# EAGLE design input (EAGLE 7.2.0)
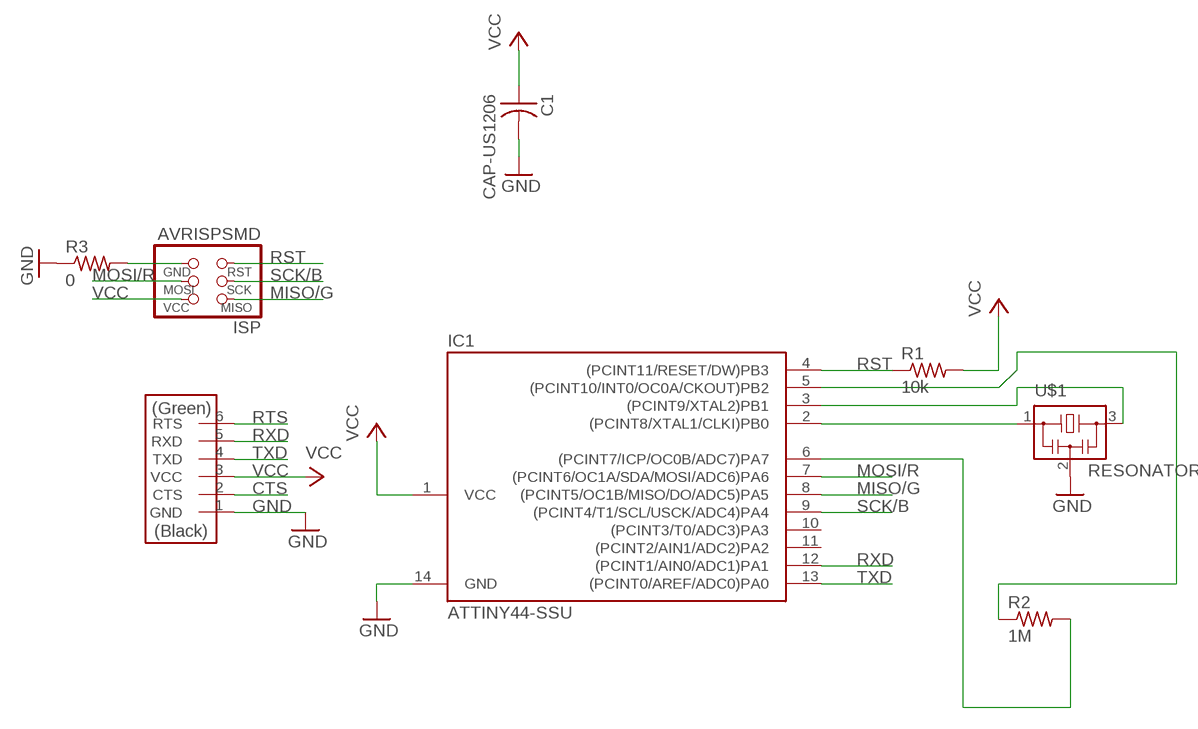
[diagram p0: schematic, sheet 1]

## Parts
C1  CAP-US1206  [C1206]
IC1  ATTINY44-SSU  [SOIC14]
ISP  AVRISPSMD  [2X03SMD]
R1  10k  RES-US1206  [R1206]
R2  1M  RES-US1206  [R1206]
R3  0  RES-US1206  [R1206]
U$1  RESONATOR  [EFOBM]
U$2  FTDI-SMD-HEADER  [1X06SMD]

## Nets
CTS: U$2.2(CTS)
GND: C1.2 IC1.14(GND) R3.1 U$1.2 U$2.1(GND)
MISO/G: IC1.8((PCINT5/OC1B/MISO/DO/ADC5)PA5) ISP.1(MISO)
MOSI/R: IC1.7((PCINT6/OC1A/SDA/MOSI/ADC6)PA6) ISP.4(MOSI)
N$1: IC1.5((PCINT10/INT0/OC0A/CKOUT)PB2) R2.1
N$2: IC1.6((PCINT7/ICP/OC0B/ADC7)PA7) R2.2
N$3: ISP.6(GND) R3.2
N$9: IC1.2((PCINT8/XTAL1/CLKI)PB0) U$1.1
N$10: IC1.3((PCINT9/XTAL2)PB1) U$1.3
RST: IC1.4((PCINT11/RESET/DW)PB3) ISP.5(RST) R1.1
RTS: U$2.6(RTS)
RXD: IC1.12((PCINT1/AIN0/ADC1)PA1) U$2.5(RXD)
SCK/B: IC1.9((PCINT4/T1/SCL/USCK/ADC4)PA4) ISP.3(SCK)
TXD: IC1.13((PCINT0/AREF/ADC0)PA0) U$2.4(TXD)
VCC: C1.1 IC1.1(VCC) ISP.2(VCC) R1.2 U$2.3(VCC)
Unconnected: IC1.10((PCINT3/T0/ADC3)PA3) IC1.11((PCINT2/AIN1/ADC2)PA2)

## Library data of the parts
C1 = fab:CAP-US
IC1 = fab:ATTINY44
ISP = fab:AVRISP
R1-R3 = fab:RES-US: Resistor (US Symbol)
U$1 = fab:RESONATOR
U$2 = fab:FTDI-SMD-HEADER

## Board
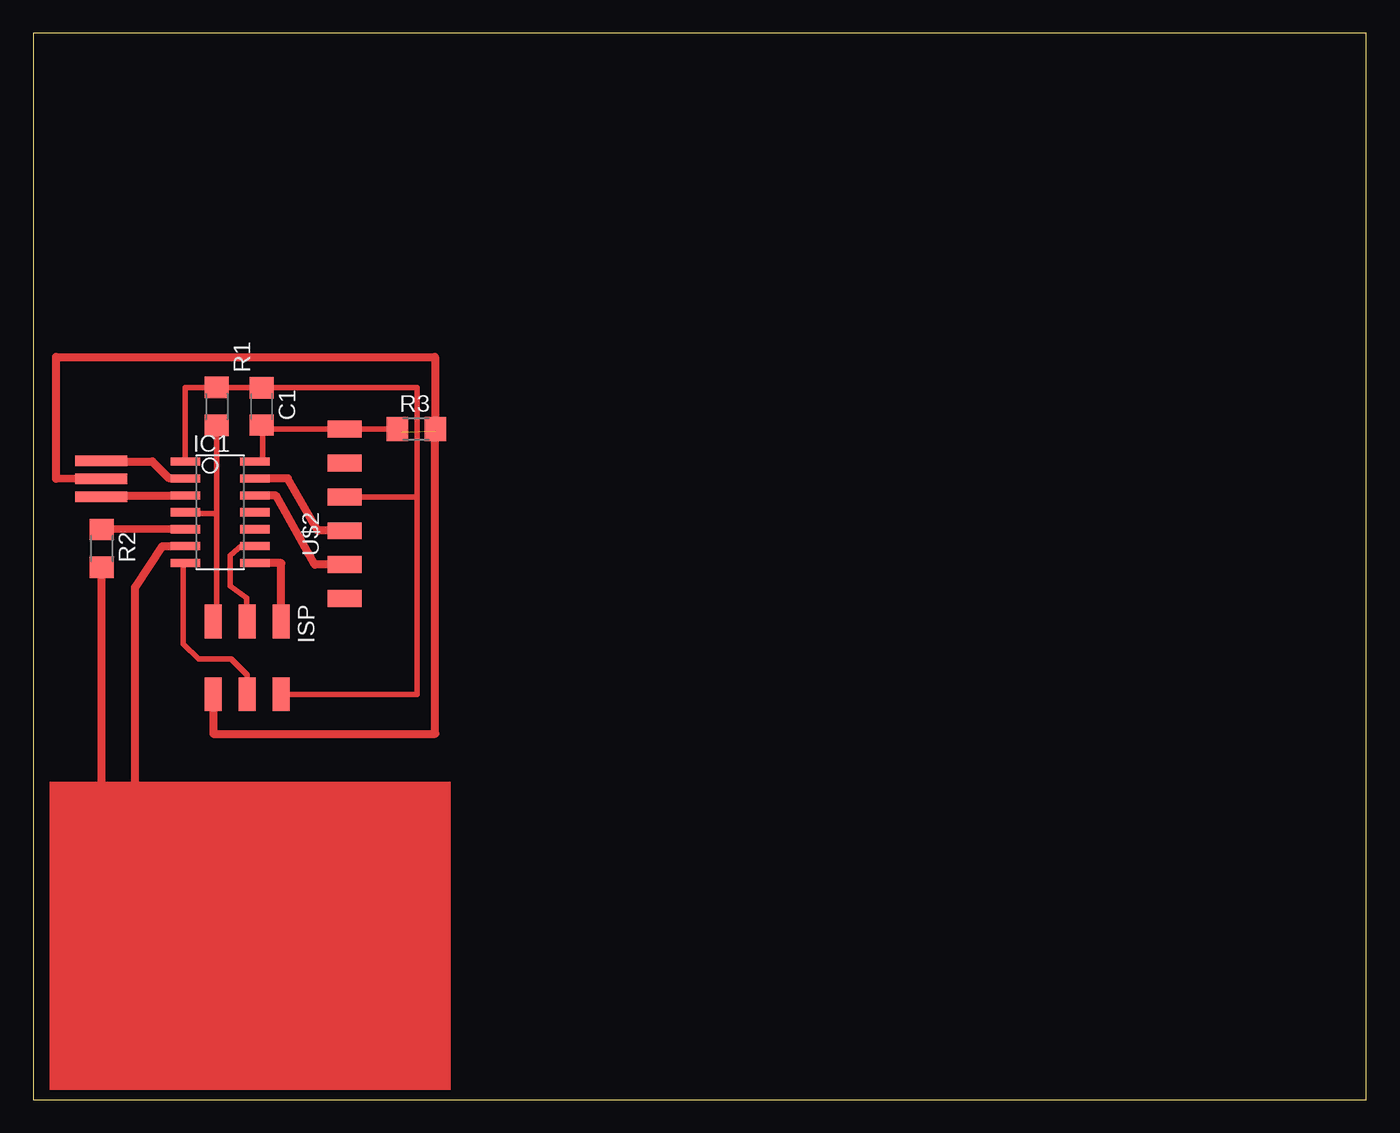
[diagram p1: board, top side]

Size 100 x 80 mm. Coordinates in mm from the lower left corner, seen from the top.
Outline: 0,0 100,0 100,80 0,80 0,0
Copper layers 1+16: Top 0.035mm / dielectric 1.5mm / Bottom 0.035mm
Design rules "fablab_17mils": minimum track width 10mil, minimum drill 0.8mm, track to track 17mil, track to pad 17mil, pad to pad 17mil, via to via 17mil, smd to smd 17mil, copper to edge 16mil, drill to drill 16mil, minimum pad ring 0.8mm, minimum via ring 0.8mm, stop-mask expansion 4mil, vias tented up to drill 0mil, thermal gap 1mm

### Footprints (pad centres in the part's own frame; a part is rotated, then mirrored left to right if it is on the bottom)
C1206 = smd 1.6 x 1.8: 1 -1.4,0; 2 1.4,0
SOIC14 = smd 0.61 x 2.21: 1 -3.81,-2.603; 2 -2.54,-2.603; 3 -1.27,-2.603; 4 0,-2.603; 5 1.27,-2.603; 6 2.54,-2.603; 7 3.81,-2.603; 8 3.81,2.603; 9 2.54,2.603; 10 1.27,2.603; 11 0,2.603; 12 -1.27,2.603; 13 -2.54,2.603; 14 -3.81,2.603
2X03SMD = smd 2.54 x 1.27: 1 -2.54,2.54; 2 2.92,2.54; 3 -2.54,0; 4 2.92,0; 5 -2.54,-2.54; 6 2.92,-2.54
R1206 = smd 1.6 x 1.803: 1 -1.422,0; 2 1.422,0
EFOBM = smd 0.8 x 3.9: 1 -1.35,0; 2 0,0; 3 1.35,0
1X06SMD = smd 2.54 x 1.27: 1 0,6.35; 2 0,3.81; 3 0,1.27; 4 0,-1.27; 5 0,-3.81; 6 0,-6.35

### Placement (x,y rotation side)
C1  17.15,52 270 top
IC1  14.02,44.06 270 top
ISP  16.05,33.33 270 top
R1  13.76,52.01 90 top
R2  5.14,41.35 270 top
R3  28.73,50.3 0 top
U$1  5.08,46.58 270 top
U$2  23.36,43.95 0 top

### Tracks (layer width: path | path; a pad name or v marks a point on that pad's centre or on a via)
GND  (1 unrouted)
  Top 0.406: C1.2 17.19,50.55 | 17.19,50.55 17.19,47.86 17.18,47.87 IC1.14 | 17.19,50.55 17.45,50.3 U$2.1 26.78,50.3 R3.1 27.64,50.09
  Top 0.61: U$1.2 1.71,46.56 1.71,55.71 30.14,55.72 30.14,50.14
MISO/G
  Top 0.406: 17.5,40.25 IC1.8
  Top 0.61: ISP.1 18.59,40.25 17.5,40.25
MOSI/R
  Top 0.406: IC1.7 11.26,40.1 11.26,34.19 12.39,33.06 14.86,33.06 16.05,31.87 ISP.4
N$1
  Top 0.61: IC1.5 R2.1
N$2
  Top 0.406: 7.67,38.47 7.62,38.43 | 7.62,22.23 5.08,22.23 5.14,22.29
  Top 0.61: 7.67,38.47 9.7,41.52 IC1.6 | 7.62,38.43 7.62,22.23 | 5.14,22.29 R2.2
N$3
  Top 0.406: ISP.6
  Top 0.61: ISP.6 13.51,27.44 30.15,27.44 R3.2
N$9
  Top 0.406: U$1.1 6.48,47.87 | 10.21,46.6 IC1.2
  Top 0.61: 6.48,47.87 8.94,47.87 10.21,46.6
N$10
  Top 0.406: U$1.3 6.48,45.33
  Top 0.61: 6.48,45.33 IC1.3
RST
  Top 0.406: R1.1 13.76,43.97 | 13.76,43.97 13.77,35.92 ISP.5 | IC1.4 11.41,43.98 13.76,43.97
RXD
  Top 0.61: U$2.5 21.11,40.14 18.22,45.31 IC1.12
SCK/B
  Top 0.406: IC1.9 16.54,41.6 15.65,41.6 14.77,40.81 14.77,38.55 16,37.64 16,35.87 ISP.3
TXD
  Top 0.61: U$2.4 21.34,42.69 19.1,46.6 IC1.13
VCC
  Top 0.406: 28.78,45.22 28.78,53.4 C1.1 13.96,53.4 R1.2 11.41,53.43 IC1.1 | 28.78,45.22 28.78,30.38 18.59,30.38 ISP.2 | U$2.3 28.78,45.22
(copper drawn outside any net)
  shapes: Top area x1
